ORGANIZATION_BLOCK MAIN:OB1
TITLE=

BEGIN
NETWORK 1
LD I1.1
O I1.2
O I1.0
ON I0.6
O I0.1
O M1.0
A I0.5
AN I0.7
AN M1.1
A I0.0
A I1.3
= M1.0

NETWORK 2
LDN I0.0
A I0.2
A I0.5
TON T37 +50

NETWORK 3
LDN I0.0
A I0.2
A I0.5
= M0.0

NETWORK 4
LD T37
O M1.1
O I0.7
AN M1.0
AN I1.0
A I0.6
A I0.2
A I0.5
AN I0.1
A I1.3
= M1.1

NETWORK 5
LD M1.0
AN I0.3
= Q0.3

NETWORK 6
LD M1.1
AN I0.4
= Q0.2
= Q0.0


NETWORK 7
LD M1.0
O M1.1
O M0.0
= Q0.6

NETWORK 8
LD SM0.5
A Q0.6
= Q0.1

NETWORK 9
LDN I0.5
= Q0.5

NETWORK 10
LD Q0.2
O Q0.3
= Q0.4

END_ORGANIZATION_BLOCK

